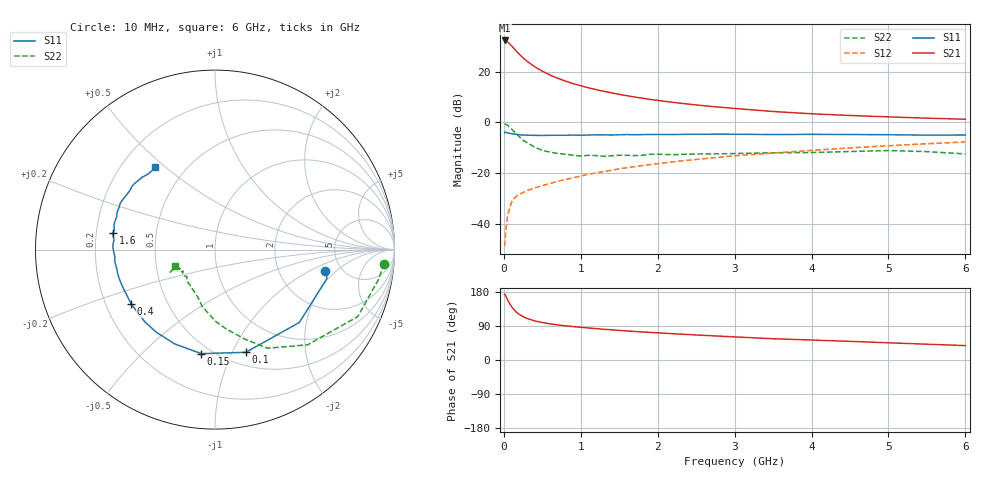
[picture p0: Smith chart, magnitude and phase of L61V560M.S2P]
!  INFINEON TECHNOLOGIES Small Signal Semiconductors
! BFR380L3 , Si-NPN RF-Transistor in TSLP-3-1
!  Vce=1.5 V,  Ic=60 mA
! Common Emitter S-Parameters:  07. March 2005
#  GHz  S  MA  R  50
! f  S11  S21  S12  S22
! GHz  Mag  Ang  Mag  Ang  Mag  Ang  Mag  Ang
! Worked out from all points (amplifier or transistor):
!   36 points, 10 MHz to 6 GHz, reference 50 ohm
!   highest |S21| = 32.4 dB at 10 MHz (marker M1)
!   |S21| within 3 dB of that: start of sweep to 126.6 MHz
!   unconditionally stable (mu >= 1): 1.312 GHz to 5.195 GHz
!   at 250 MHz: K = 0.49, MSG = 26.6 dB, |S12| = -27.7 dB
!   at 1.4 GHz: K = 1.01, MAG = 14.7 dB, |S12| = -18.9 dB
!   at 6 GHz: K = 0.99, MSG = 4.5 dB, |S12| = -7.7 dB
!   S11 on the Smith chart (normalised r, x): 10 MHz: 3.71, -1.48; 100 MHz: 0.63, -1.13; 150 MHz: 0.44, -0.78; 400 MHz: 0.31, -0.27; 1.6 GHz: 0.27, +0.08; 6 GHz: 0.34, +0.46
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0.01  0.6252 -11.2  41.64 173.8  0.0036 72.3  0.9446 -4.8
0.02  0.6447 -14.3  41.29 171.3  0.006 83.1  0.9263 -10.3
0.05  0.6211 -40.8  38.85 158.1  0.0149 72.0  0.8789 -25.1
0.1  0.5974 -73.3  32.71 140.9  0.0266 60.2  0.7401 -45.8
0.15  0.5847 -97.5  26.9 128.6  0.0335 54.7  0.6229 -61.9
0.2  0.5714 -113.2  22.3 120.3  0.0383 52.2  0.5238 -71.8
0.25  0.5647 -125.3  18.91 114.4  0.0411 50.8  0.4455 -82.1
0.3  0.5611 -134.2  16.22 109.8  0.0452 50.4  0.4013 -89.3
0.4  0.5565 -147.0  12.63 103.2  0.0508 51.8  0.3262 -102.4
0.5  0.5535 -155.4  10.3 98.9  0.0567 53.8  0.2812 -109.9
0.6  0.5568 -161.2  8.62 95.4  0.0621 55.5  0.2594 -117.2
0.7  0.5584 -165.6  7.467 92.7  0.0688 57.7  0.2439 -124.1
0.9  0.5629 -173.7  5.845 88.2  0.0804 60.1  0.2248 -134.6
1.1  0.5641 -178.6  4.834 84.4  0.0949 62.0  0.2245 -139.3
1.3  0.5684 176.3  4.128 81.0  0.1078 63.3  0.215 -146.5
1.6  0.5766 170.5  3.372 76.6  0.1275 64.3  0.2247 -151.6
2.2  0.5773 161.8  2.494 69.3  0.1668 64.8  0.2307 -152.7
2.8  0.5878 153.8  2.007 63.0  0.2052 64.7  0.2405 -157.0
3.5  0.5771 145.5  1.645 56.1  0.2489 62.5  0.2519 -155.3
4.5  0.5779 139.3  1.373 49.2  0.3138 60.4  0.2665 -154.2
5.5  0.5617 131.1  1.215 41.7  0.3796 56.3  0.265 -154.3
6  0.5654 126.0  1.158 38.0  0.4123 53.9  0.2393 -158.1
